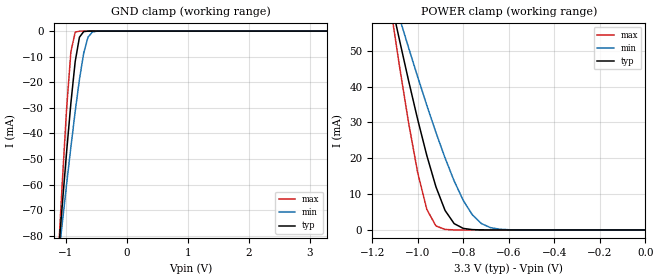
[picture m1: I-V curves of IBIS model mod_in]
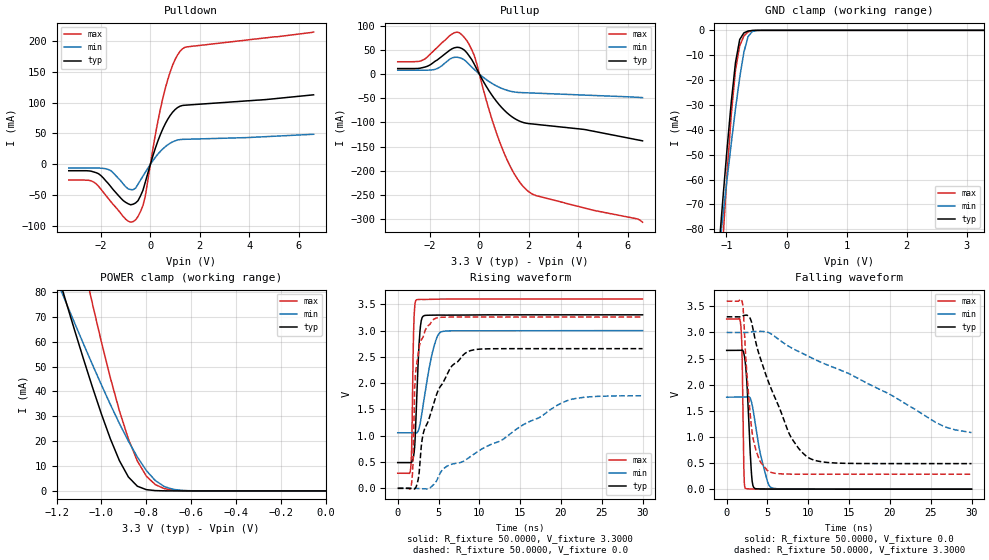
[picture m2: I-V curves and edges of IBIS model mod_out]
| IBIS (I/O, Buffer, Information, Specification) Model, officially
| electronic behavioral standard for Buffer structures of digital pins.
[IBIS ver]  4.0
[File name] 54ac16244_3v3_rev1.ibs
[File Rev]  1.0
[Date]   26 June 2020
[Source]   CAD & Design Services (Catania) - STMicroelectronics
[Notes]
  (Note1) This IBIS model is the model of the product with package
   (Flat48 package elements);
  (Note2) This IBIS model is extracted with nominal 3.3V power supply
   (min:3.0V, typ:3.3V, max:3.6V);
  (Note3) This model has few Warnings about the non-monotonicity
   of I-V curves, but they are not indicative of problems
   inside the model;
[Copyright] (c) 2020 STMicroelectronics
|   Component 54AC16244
[Component] 54AC16244
[Manufacturer] STMicroelectronics
[Package]
| variable  typ   min   max
R_pkg   0.0   0.0   0.0
L_pkg   0.0H   0.0H   0.0H
C_pkg   0.0F   0.0F   0.0F
[Pin]  signal_name   model_name   R_pin   L_pin   C_pin
1   N1GN   mod_in   467.00m   6.34nH   1.49pF
2   N1Y1   mod_out   467.00m   6.34nH   1.49pF
3   N1Y2   mod_out   467.00m   6.34nH   1.49pF
4   GND1   GND   467.00m   6.34nH   1.49pF
5   N1Y3   mod_out   145.00m   3.32nH   1.24pF
6   N1Y4   mod_out   141.00m   2.11nH   1.24pF
7   VCC1   POWER   141.00m   2.11nH   1.24pF
8   N2Y1   mod_out   141.00m   2.11nH   1.24pF
9   N2Y2   mod_out   141.00m   2.11nH   1.24pF
10   GND2   GND   141.00m   2.11nH   1.24pF
11   N2Y3   mod_out   141.00m   2.11nH   1.24pF
12   N2Y4   mod_out   141.00m   2.11nH   1.24pF
13   N3Y1   mod_out   141.00m   2.11nH   1.24pF
14   N3Y2   mod_out   141.00m   2.11nH   1.24pF
15   GND3   GND   141.00m   2.11nH   1.24pF
16   N3Y3   mod_out   141.00m   2.11nH   1.24pF
17   N3Y4   mod_out   141.00m   2.11nH   1.24pF
18   VCC2   POWER   141.00m   2.11nH   1.24pF
19   N4Y1   mod_out   141.00m   2.11nH   1.24pF
20   N4Y2   mod_out   145.00m   3.32nH   1.24pF
21   GND4   GND   467.00m   6.34nH   1.49pF
22   N4Y3   mod_out   467.00m   6.34nH   1.49pF
23   N4Y4   mod_out   467.00m   6.34nH   1.49pF
24   N4GN   mod_in   467.00m   6.34nH   1.49pF
25   N3GN   mod_in   467.00m   6.34nH   1.49pF
26   N4A4   mod_in   467.00m   6.34nH   1.49pF
27   N4A3   mod_in   467.00m   6.34nH   1.49pF
28   GND5   GND   467.00m   6.34nH   1.49pF
29   N4A2   mod_in   145.00m   3.32nH   1.24pF
30   N4A1   mod_in   141.00m   2.11nH   1.24pF
31   VCC3   POWER   141.00m   2.11nH   1.24pF
32   N3A4   mod_in   141.00m   2.11nH   1.24pF
33   N3A3   mod_in   141.00m   2.11nH   1.24pF
34   GND6   GND   141.00m   2.11nH   1.24pF
35   N3A2   mod_in   141.00m   2.11nH   1.24pF
36   N3A1   mod_in   141.00m   2.11nH   1.24pF
37   N2A4   mod_in   141.00m   2.11nH   1.24pF
38   N2A3   mod_in   141.00m   2.11nH   1.24pF
39   GND7   GND   141.00m   2.11nH   1.24pF
40   N2A2   mod_in   141.00m   2.11nH   1.24pF
41   N2A1   mod_in   141.00m   2.11nH   1.24pF
42   VCC4   POWER   141.00m   2.11nH   1.24pF
43   N1A4   mod_in   141.00m   2.11nH   1.24pF
44   N1A3   mod_in   145.00m   3.32nH   1.24pF
45   GND8   GND   467.00m   6.34nH   1.49pF
46   N1A2   mod_in   467.00m   6.34nH   1.49pF
47   N1A1   mod_in   467.00m   6.34nH   1.49pF
48   N2GN   mod_in   467.00m   6.34nH   1.49pF
| Models and submodels in the file (2): mod_in (Input), mod_out (3-state)
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|   Model mod_in
[Model]   mod_in
Model_type Input
Vinl   =   1.000V
Vinh   =   2.300V
C_comp   0.584pF   0.476pF   0.722pF
[Temperature Range]  25.0000   0.1250k   -55.0000
[Voltage Range]   3.3000V   3.0000V   3.6000V
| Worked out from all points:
|   GND clamp passes 1 mA (typ) near -0.74 V on its own axis
|   POWER clamp passes 1 mA (typ) near -0.82 V on its own axis
[GND_clamp]
|Voltage   I(typ)   I(min)   I(max)
-3.3V     -798.8mA   -595.3mA   -1.138A
-1.13V    -88.7mA    -90.03mA   -89.3mA
-1.06V    -67.54mA   -74.76mA   -58.64mA
-990mV    -47.13mA   -59.8mA    -30.22mA
-920mV    -28.09mA   -45.3mA    -8.012mA
-850mV    -11.96mA   -31.49mA   -440.9uA
-780mV    -2.392mA   -18.91mA   -11.16uA
-710mV    -202.9uA   -8.609mA   -269.9nA
-640mV    -13.61uA   -2.392mA   -6.525nA
-570mV    -893.7nA   -397.5uA   -166.8pA
-430mV    -3.851nA   -7.049uA   -9.012pA
3.28V     6.52pA     5.985nA    5.92pA
[POWER_clamp]
|Voltage   I(typ)   I(min)   I(max)
-3.28V    769.1mA    568.6mA    1.103A
-1.12V    64.69mA    67.68mA    62.53mA
-1.08V    52.98mA    59.19mA    45.69mA
-1.04V    41.63mA    50.84mA    29.88mA
-1V       30.8mA     42.69mA    15.96mA
-960mV    20.77mA    34.78mA    5.737mA
-920mV    12.05mA    27.21mA    1.129mA
-880mV    5.461mA    20.1mA     149.7uA
-840mV    1.772mA    13.68mA    18.09uA
-760mV    95.93uA    4.215mA    257.2nA
-680mV    4.309uA    635.2uA    3.657nA
0V        6.6pA      45.39pA    7.2pA
|   Model mod_out
[Model]   mod_out
Model_type 3-state
Polarity   Non-Inverting
Enable   Active-Low
Vmeas  =   1.650V
Cref   =   50pF
Rref   =   500
C_comp   3.063pF   2.328pF   4.030pF
[Temperature Range]  25.0000   0.1250k   -55.0000
[Voltage Range]   3.3000V   3.0000V   3.6000V
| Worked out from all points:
|   slope of the pulldown table from 0 to 0.495 V, typ, clamps not added: 8.73 ohm
|   slope of the pullup table from 0 to 0.495 V, typ, clamps not added: 11.6 ohm
|   GND clamp passes 1 mA (typ) near -0.71 V on its own axis
|   POWER clamp passes 1 mA (typ) near -0.81 V on its own axis
|   rising waveform, R_fixture 50.0000, V_fixture 3.3000: 20-80 % time 452ps typ, 1.31ns min, 209ps max; typ from 0.489 V to 3.3 V
|   rising waveform, R_fixture 50.0000, V_fixture 0.0: 20-80 % time 3.19ns typ, 12.5ns min, 655ps max; typ from 0 V to 2.66 V
|   falling waveform, R_fixture 50.0000, V_fixture 0.0: 20-80 % time 502ps typ, 1.3ns min, 195ps max; typ from 2.66 V to 0 V
|   falling waveform, R_fixture 50.0000, V_fixture 3.3000: 20-80 % time 4.01ns typ, 14.6ns min, 1.08ns max; typ from 3.3 V to 0.489 V
[Pulldown]
|Voltage   I(typ)   I(min)   I(max)
-3.3V     -10.36mA   -6mA       -25.42mA
-2.3V     -12.22mA   -6mA       -28.55mA
-1.6V     -36.13mA   -10.2mA    -60.32mA
-1V       -61.53mA   -36.2mA    -88.81mA
-700mV    -64.64mA   -41.15mA   -92.74mA
-300mV    -42.01mA   -19.04mA   -66.8mA
-200mV    -28.05mA   -12.57mA   -50.55mA
200mV     25.93mA    11.34mA    47.73mA
500mV     57.16mA    24.87mA    106.4mA
900mV     84.46mA    36.38mA    160.6mA
1.2V      94.2mA     40.13mA    183.1mA
6.6V      112.6mA    48.7mA     214.2mA
[Pullup]
|Voltage   I(typ)   I(min)   I(max)
-3.3V     11.36mA    8mA        25.42mA
-2.3V     13.22mA    8mA        28.55mA
-1.7V     29.13mA    11.44mA    55.32mA
-1.2V     49.14mA    30.66mA    79.32mA
-800mV    54.74mA    33.68mA    85.2mA
-500mV    43.64mA    24.28mA    68.7mA
-200mV    19.98mA    9.243mA    37.72mA
400mV     -35.28mA   -15.69mA   -75.16mA
1V        -74.32mA   -31.52mA   -163.1mA
1.8V      -100.5mA   -38.51mA   -233.9mA
2.3V      -104mA     -39.52mA   -251.2mA
6.6V      -138mA     -48.7mA    -306.1mA
[GND_clamp]
|Voltage   I(typ)   I(min)   I(max)
-3.3V     -798.9mA   -595.3mA   -1.148A
-1.13V    -89mA      -90.08mA   -113.7mA
-1.06V    -67.9mA    -74.82mA   -84.69mA
-990mV    -47.6mA    -59.87mA   -57.63mA
-920mV    -28.75mA   -45.37mA   -33.93mA
-850mV    -12.97mA   -31.59mA   -16.07mA
-780mV    -3.71mA    -19.02mA   -6.223mA
-710mV    -1.021mA   -8.74mA    -2.256mA
-640mV    -262.7uA   -2.504mA   -623.3uA
-570mV    -57.33uA   -455.2uA   -83.11uA
-500mV    -11.95uA   -74.74uA   -9.782uA
3.28V     84.16pA    10.71nA    15.02pA
[POWER_clamp]
|Voltage   I(typ)   I(min)   I(max)
-3.28V    769.1mA    568.6mA    1.132A
-1.2V     88.92mA    84.99mA    142.3mA
-1.16V    76.76mA    76.28mA    125mA
-1.08V    53.09mA    59.17mA    91.37mA
-1.04V    41.75mA    50.82mA    75.3mA
-920mV    12.22mA    27.17mA    32.3mA
-880mV    5.633mA    20.07mA    20.96mA
-840mV    1.905mA    13.64mA    12.05mA
-800mV    513.7uA    8.218mA    5.986mA
-760mV    132.7uA    4.183mA    2.534mA
-640mV    3.963uA    205.9uA    111.1uA
0V        86.27pA    0A         22.24pA
[Ramp]
| variable   typ   min   max
dV/dt_r   1.5938/3.1727n   1.0567/12.4426n   1.9547/0.6804n
dV/dt_f   1.6861/4.0132n   1.1225/14.4411n   1.9881/1.0738n
R_load = 50.0000
[Rising Waveform]
R_fixture= 50.0000
V_fixture= 3.3000
V_fixture_min= 3.0000
V_fixture_max= 3.6000
|time   V(typ)   V(min)   V(max)
0s        489.4mV    1.057V     286.6mV
1.59ns    487.8mV    1.057V     383.2mV
1.71ns    496.3mV    1.057V     773mV
1.95ns    618.2mV    1.057V     3.012V
2.31ns    1.648V     1.054V     3.586V
2.67ns    2.875V     1.173V     3.593V
2.97ns    3.239V     1.435V     3.594V
4.23ns    3.294V     2.572V     3.595V
5.31ns    3.295V     2.975V     3.599V
30ns      3.3V       3V         3.6V
[Rising Waveform]
R_fixture= 50.0000
V_fixture= 0.0
V_fixture_min= 0.0
V_fixture_max= 0.0
|time   V(typ)   V(min)   V(max)
0s        132.2pV    0V         79.8pV
1.59ns    -268.4uV   -29.46uV   7.888mV
1.86ns    -11.53mV   234.2uV    428mV
2.07ns    -11.04mV   670.4uV    1.854V
2.28ns    37.71mV    -863.9uV   2.316V
3.12ns    1.038V     -9.771mV   2.885V
4.44ns    1.631V     76.98mV    3.218V
9.06ns    2.625V     620.2mV    3.258V
20.7ns    2.657V     1.664V     3.258V
30ns      2.657V     1.761V     3.258V
[Falling Waveform]
R_fixture= 50.0000
V_fixture= 0.0
V_fixture_min= 0.0
V_fixture_max= 0.0
|time   V(typ)   V(min)   V(max)
0s        2.657V     1.762V     3.258V
1.68ns    2.656V     1.761V     3.204V
1.86ns    2.662V     1.761V     2.762V
2.1ns     2.601V     1.761V     411.4mV
2.28ns    2.426V     1.762V     16.55mV
3.06ns    255.5mV    1.659V     2.864mV
3.42ns    17.11mV    1.335V     3.371mV
4.86ns    2.283mV    217.9mV    2.06mV
5.58ns    1.624mV    23.03mV    1.039mV
30ns      -218.4nV   205.4uV    -911.9nV
[Falling Waveform]
R_fixture= 50.0000
V_fixture= 3.3000
V_fixture_min= 3.0000
V_fixture_max= 3.6000
|time   V(typ)   V(min)   V(max)
0s        3.3V       3V         3.6V
1.89ns    3.305V     3V         3.594V
2.01ns    3.32V      3V         3.478V
2.52ns    3.328V     2.999V     2.123V
3.12ns    3.148V     3.015V     1.082V
4.02ns    2.555V     3.021V     558.5mV
5.04ns    2.085V     3.005V     352.3mV
7.86ns    1.002V     2.712V     287.8mV
10.41ns   572.6mV    2.513V     286.7mV
30ns      489.4mV    1.083V     286.6mV
